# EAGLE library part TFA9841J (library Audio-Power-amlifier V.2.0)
The TFA9841J contains one audio power amplifier. The TFA9841J can be used as one Single-Ended (SE) channel with a fixed gain of 26 dB. The TFA9841J comes in a 9-pin DIL-bent-SIL (DBS9P) power package. The TFA9841J is pin compatible with the TFA9842J and TFA9843J. The TFA9841J contains a unique protection circuit that is solely based on multiple temperature measurements inside the chip. This gives maximum output power for all supply voltages and load conditions with no unnecessary audio holes. Almost any supply voltage and load impedance combination can be made as long as thermal boundary conditions (external heatsink and ambient temperature) allow it.
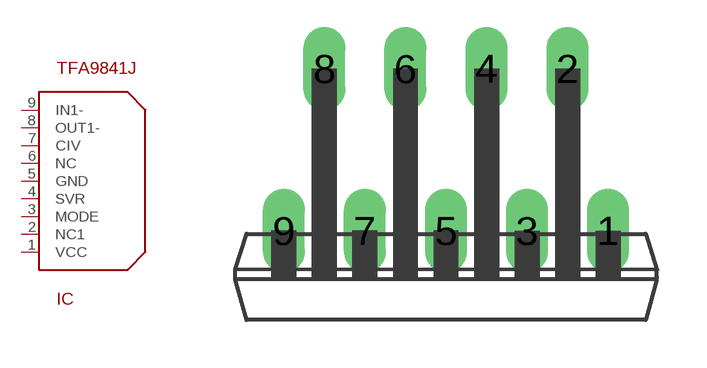
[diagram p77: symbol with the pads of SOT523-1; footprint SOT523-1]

Designator prefix IC

## TFA9841J  [SOT523-1]
1  VCC  pwr
2  NC1  out
3  MODE
4  SVR
5  GND  pwr
6  NC  in
7  CIV
8  OUT1-  out
9  IN1-  in

## Footprint SOT523-1 (pad centres in mm)
drill 0.8 long: 1 5.08,0; 2 3.81,5.08; 3 2.54,0; 4 1.27,5.08; 5 0,0; 6 -1.27,5.08; 7 -2.54,0; 8 -3.81,5.08; 9 -5.08,0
